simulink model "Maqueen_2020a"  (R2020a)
settings: Solver=VariableStepAuto  StartTime=0.0  StopTime=2  RelTol=1e-3
model workspace: external: MAT-File (data not in the file)
undefined symbols (not defined in the file or in its folder): deg, kg, m, mm, N, rad, s, smiData, X, Y, Z
libraries: sm_lib x459, fl_lib x12, nesl_utility x10
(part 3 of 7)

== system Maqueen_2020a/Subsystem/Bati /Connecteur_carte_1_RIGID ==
  ReferenceFrame : sm_lib/Frames and Transforms/Reference Frame
  Solid : sm_lib/Body Elements/File Solid  ExtGeomFileName=Connecteur carte_Defaut_sldprt.STL  UnitType=Custom  ExtGeomFileUnits=mm  StepReaderType=HEX  ExportConvexHullGeometry=off  InertiaType=Custom  Mass=smiData.Solid(28).mass  MassUnits=kg  CenterOfMass=smiData.Solid(28).CoM  CenterOfMassUnits=mm  MomentsOfInertia=smiData.Solid(28).MoI  MomentsOfInertiaUnits=kg*mm^2  ProductsOfInertia=smiData.Solid(28).PoI  ProductsOfInertiaUnits=kg*mm^2  BasedOnType=Density  Density=1000  DensityUnits=kg/m^3  DoExposeReferenceFrame=on  SerializedFrames=<Frames/>  GraphicType=FromGeometry  MarkerShape=Sphere  MarkerSize=10  GraphicVisPropType=SimpleVisualProperties  GraphicDiffuseColor=smiData.Solid(28).color  GraphicSpecularColor=[0.5 0.5 0.5 1.0]  GraphicAmbientColor=[0.15 0.15 0.15 1.0]  GraphicEmissiveColor=[0.0 0.0 0.0 1.0]  GraphicShininess=75  GraphicOpacity=smiData.Solid(28).opacity
  Transform : sm_lib/Frames and Transforms/Rigid Transform  TranslationMethod=Cartesian  TranslationStandardOffset=0  TranslationLengthUnit=mm  TranslationStandardAxis=+Z  TranslationCartesianOffset=smiData.RigidTransform(4).translation  TranslationROffset=0  TranslationROffsetUnits=m  TranslationZOffset=0  TranslationZOffsetUnits=m  TranslationThetaOffset=0  TranslationThetaOffsetUnits=deg  RotationMethod=ArbitraryAxis  RotationAngleUnits=rad  RotationStandardAxis=+Z  RotationAngle=smiData.RigidTransform(4).angle  RotationArbitraryAxis=smiData.RigidTransform(4).axis  FollAlignAxisA=+X  BaseAlignAxisA=+Y  FollAlignAxisB=+Y  BaseAlignAxisB=+Z  RotationSequenceAxes=FollowerAxes  RotationSequence=XYX  RotationSequenceAngles=[0 0 0]  RotationSequenceAnglesUnits=deg  RotationMatrix=[1 0 0; 0 1 0; 0 0 1]
  Transform1 : sm_lib/Frames and Transforms/Rigid Transform  TranslationMethod=Cartesian  TranslationStandardOffset=0  TranslationLengthUnit=mm  TranslationStandardAxis=+Z  TranslationCartesianOffset=smiData.RigidTransform(5).translation  TranslationROffset=0  TranslationROffsetUnits=m  TranslationZOffset=0  TranslationZOffsetUnits=m  TranslationThetaOffset=0  TranslationThetaOffsetUnits=deg  RotationMethod=ArbitraryAxis  RotationAngleUnits=rad  RotationStandardAxis=+Z  RotationAngle=smiData.RigidTransform(5).angle  RotationArbitraryAxis=smiData.RigidTransform(5).axis  FollAlignAxisA=+X  BaseAlignAxisA=+Y  FollAlignAxisB=+Y  BaseAlignAxisB=+Z  RotationSequenceAxes=FollowerAxes  RotationSequence=XYX  RotationSequenceAngles=[0 0 0]  RotationSequenceAnglesUnits=deg  RotationMatrix=[1 0 0; 0 1 0; 0 0 1]
  F : PMIOPort  Side=Left
  F1 : PMIOPort  Port=2  Side=Left
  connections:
  ReferenceFrame/RConn1 -- Transform/LConn1 -- Transform1/LConn1 -- Solid/RConn1
  Transform/RConn1 -- F/RConn1
  Transform1/RConn1 -- F1/RConn1

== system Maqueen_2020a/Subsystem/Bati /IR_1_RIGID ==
  ReferenceFrame : sm_lib/Frames and Transforms/Reference Frame
  Solid : sm_lib/Body Elements/File Solid  ExtGeomFileName=IR_Defaut_sldprt.STL  UnitType=Custom  ExtGeomFileUnits=mm  StepReaderType=HEX  ExportConvexHullGeometry=off  InertiaType=Custom  Mass=smiData.Solid(32).mass  MassUnits=kg  CenterOfMass=smiData.Solid(32).CoM  CenterOfMassUnits=mm  MomentsOfInertia=smiData.Solid(32).MoI  MomentsOfInertiaUnits=kg*mm^2  ProductsOfInertia=smiData.Solid(32).PoI  ProductsOfInertiaUnits=kg*mm^2  BasedOnType=Density  Density=1000  DensityUnits=kg/m^3  DoExposeReferenceFrame=on  SerializedFrames=<Frames/>  GraphicType=FromGeometry  MarkerShape=Sphere  MarkerSize=10  GraphicVisPropType=SimpleVisualProperties  GraphicDiffuseColor=smiData.Solid(32).color  GraphicSpecularColor=[0.5 0.5 0.5 1.0]  GraphicAmbientColor=[0.15 0.15 0.15 1.0]  GraphicEmissiveColor=[0.0 0.0 0.0 1.0]  GraphicShininess=75  GraphicOpacity=smiData.Solid(32).opacity
  Transform : sm_lib/Frames and Transforms/Rigid Transform  TranslationMethod=Cartesian  TranslationStandardOffset=0  TranslationLengthUnit=mm  TranslationStandardAxis=+Z  TranslationCartesianOffset=smiData.RigidTransform(10).translation  TranslationROffset=0  TranslationROffsetUnits=m  TranslationZOffset=0  TranslationZOffsetUnits=m  TranslationThetaOffset=0  TranslationThetaOffsetUnits=deg  RotationMethod=ArbitraryAxis  RotationAngleUnits=rad  RotationStandardAxis=+Z  RotationAngle=smiData.RigidTransform(10).angle  RotationArbitraryAxis=smiData.RigidTransform(10).axis  FollAlignAxisA=+X  BaseAlignAxisA=+Y  FollAlignAxisB=+Y  BaseAlignAxisB=+Z  RotationSequenceAxes=FollowerAxes  RotationSequence=XYX  RotationSequenceAngles=[0 0 0]  RotationSequenceAnglesUnits=deg  RotationMatrix=[1 0 0; 0 1 0; 0 0 1]
  F : PMIOPort  Side=Left
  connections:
  ReferenceFrame/RConn1 -- Solid/RConn1 -- Transform/LConn1
  Transform/RConn1 -- F/RConn1

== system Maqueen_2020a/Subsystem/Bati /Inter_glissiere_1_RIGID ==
  ReferenceFrame : sm_lib/Frames and Transforms/Reference Frame
  Solid : sm_lib/Body Elements/File Solid  ExtGeomFileName=Inter_glissiere_Defaut_sldprt.STL  UnitType=Custom  ExtGeomFileUnits=mm  StepReaderType=HEX  ExportConvexHullGeometry=off  InertiaType=Custom  Mass=smiData.Solid(1).mass  MassUnits=kg  CenterOfMass=smiData.Solid(1).CoM  CenterOfMassUnits=mm  MomentsOfInertia=smiData.Solid(1).MoI  MomentsOfInertiaUnits=kg*mm^2  ProductsOfInertia=smiData.Solid(1).PoI  ProductsOfInertiaUnits=kg*mm^2  BasedOnType=Density  Density=1000  DensityUnits=kg/m^3  DoExposeReferenceFrame=on  SerializedFrames=<Frames/>  GraphicType=FromGeometry  MarkerShape=Sphere  MarkerSize=10  GraphicVisPropType=SimpleVisualProperties  GraphicDiffuseColor=smiData.Solid(1).color  GraphicSpecularColor=[0.5 0.5 0.5 1.0]  GraphicAmbientColor=[0.15 0.15 0.15 1.0]  GraphicEmissiveColor=[0.0 0.0 0.0 1.0]  GraphicShininess=75  GraphicOpacity=smiData.Solid(1).opacity
  Transform : sm_lib/Frames and Transforms/Rigid Transform  TranslationMethod=Cartesian  TranslationStandardOffset=0  TranslationLengthUnit=mm  TranslationStandardAxis=+Z  TranslationCartesianOffset=smiData.RigidTransform(12).translation  TranslationROffset=0  TranslationROffsetUnits=m  TranslationZOffset=0  TranslationZOffsetUnits=m  TranslationThetaOffset=0  TranslationThetaOffsetUnits=deg  RotationMethod=ArbitraryAxis  RotationAngleUnits=rad  RotationStandardAxis=+Z  RotationAngle=smiData.RigidTransform(12).angle  RotationArbitraryAxis=smiData.RigidTransform(12).axis  FollAlignAxisA=+X  BaseAlignAxisA=+Y  FollAlignAxisB=+Y  BaseAlignAxisB=+Z  RotationSequenceAxes=FollowerAxes  RotationSequence=XYX  RotationSequenceAngles=[0 0 0]  RotationSequenceAnglesUnits=deg  RotationMatrix=[1 0 0; 0 1 0; 0 0 1]
  F : PMIOPort  Side=Left
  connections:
  ReferenceFrame/RConn1 -- Solid/RConn1 -- Transform/LConn1
  Transform/RConn1 -- F/RConn1

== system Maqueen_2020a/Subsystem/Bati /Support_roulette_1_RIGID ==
  ReferenceFrame : sm_lib/Frames and Transforms/Reference Frame
  Rouleau_1_RIGID : Subsystem
  Support_roulette_1_RIGID : Subsystem
  Transform : sm_lib/Frames and Transforms/Rigid Transform  TranslationMethod=Cartesian  TranslationStandardOffset=0  TranslationLengthUnit=mm  TranslationStandardAxis=+Z  TranslationCartesianOffset=smiData.RigidTransform(8).translation  TranslationROffset=0  TranslationROffsetUnits=m  TranslationZOffset=0  TranslationZOffsetUnits=m  TranslationThetaOffset=0  TranslationThetaOffsetUnits=deg  RotationMethod=ArbitraryAxis  RotationAngleUnits=rad  RotationStandardAxis=+Z  RotationAngle=smiData.RigidTransform(8).angle  RotationArbitraryAxis=smiData.RigidTransform(8).axis  FollAlignAxisA=+X  BaseAlignAxisA=+Y  FollAlignAxisB=+Y  BaseAlignAxisB=+Z  RotationSequenceAxes=FollowerAxes  RotationSequence=XYX  RotationSequenceAngles=[0 0 0]  RotationSequenceAnglesUnits=deg  RotationMatrix=[1 0 0; 0 1 0; 0 0 1]
  Transform1 : sm_lib/Frames and Transforms/Rigid Transform  TranslationMethod=Cartesian  TranslationStandardOffset=0  TranslationLengthUnit=mm  TranslationStandardAxis=+Z  TranslationCartesianOffset=smiData.RigidTransform(159).translation  TranslationROffset=0  TranslationROffsetUnits=m  TranslationZOffset=0  TranslationZOffsetUnits=m  TranslationThetaOffset=0  TranslationThetaOffsetUnits=deg  RotationMethod=ArbitraryAxis  RotationAngleUnits=rad  RotationStandardAxis=+Z  RotationAngle=smiData.RigidTransform(159).angle  RotationArbitraryAxis=smiData.RigidTransform(159).axis  FollAlignAxisA=+X  BaseAlignAxisA=+Y  FollAlignAxisB=+Y  BaseAlignAxisB=+Z  RotationSequenceAxes=FollowerAxes  RotationSequence=XYX  RotationSequenceAngles=[0 0 0]  RotationSequenceAnglesUnits=deg  RotationMatrix=[1 0 0; 0 1 0; 0 0 1]
  Transform2 : sm_lib/Frames and Transforms/Rigid Transform  TranslationMethod=Cartesian  TranslationStandardOffset=0  TranslationLengthUnit=mm  TranslationStandardAxis=+Z  TranslationCartesianOffset=smiData.RigidTransform(160).translation  TranslationROffset=0  TranslationROffsetUnits=m  TranslationZOffset=0  TranslationZOffsetUnits=m  TranslationThetaOffset=0  TranslationThetaOffsetUnits=deg  RotationMethod=ArbitraryAxis  RotationAngleUnits=rad  RotationStandardAxis=+Z  RotationAngle=smiData.RigidTransform(160).angle  RotationArbitraryAxis=smiData.RigidTransform(160).axis  FollAlignAxisA=+X  BaseAlignAxisA=+Y  FollAlignAxisB=+Y  BaseAlignAxisB=+Z  RotationSequenceAxes=FollowerAxes  RotationSequence=XYX  RotationSequenceAngles=[0 0 0]  RotationSequenceAnglesUnits=deg  RotationMatrix=[1 0 0; 0 1 0; 0 0 1]
  F : PMIOPort  Side=Left
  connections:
  ReferenceFrame/RConn1 -- Transform/LConn1 -- Transform1/LConn1 -- Transform2/LConn1
  Transform/RConn1 -- F/RConn1
  Support_roulette_1_RIGID/LConn1 -- Transform1/RConn1
  Rouleau_1_RIGID/LConn1 -- Transform2/RConn1

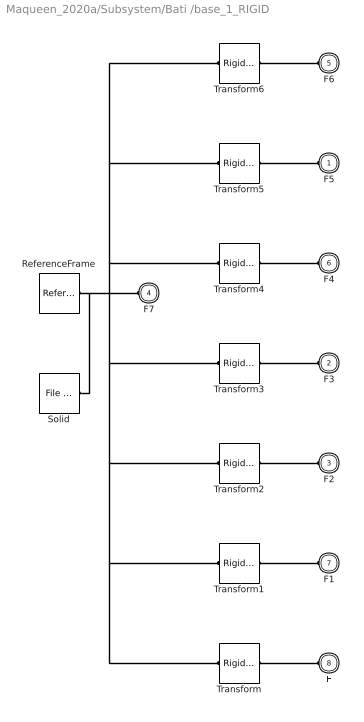
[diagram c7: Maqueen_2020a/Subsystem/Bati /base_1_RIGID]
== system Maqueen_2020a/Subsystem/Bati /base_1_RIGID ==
  ReferenceFrame : sm_lib/Frames and Transforms/Reference Frame
  Solid : sm_lib/Body Elements/File Solid  ExtGeomFileName=base_Defaut_sldprt.STL  UnitType=Custom  ExtGeomFileUnits=mm  StepReaderType=HEX  ExportConvexHullGeometry=off  InertiaType=Custom  Mass=smiData.Solid(29).mass  MassUnits=kg  CenterOfMass=smiData.Solid(29).CoM  CenterOfMassUnits=mm  MomentsOfInertia=smiData.Solid(29).MoI  MomentsOfInertiaUnits=kg*mm^2  ProductsOfInertia=smiData.Solid(29).PoI  ProductsOfInertiaUnits=kg*mm^2  BasedOnType=Density  Density=1000  DensityUnits=kg/m^3  DoExposeReferenceFrame=on  SerializedFrames=<Frames/>  GraphicType=FromGeometry  MarkerShape=Sphere  MarkerSize=10  GraphicVisPropType=SimpleVisualProperties  GraphicDiffuseColor=smiData.Solid(29).color  GraphicSpecularColor=[0.5 0.5 0.5 1.0]  GraphicAmbientColor=[0.15 0.15 0.15 1.0]  GraphicEmissiveColor=[0.0 0.0 0.0 1.0]  GraphicShininess=75  GraphicOpacity=smiData.Solid(29).opacity
  Transform : sm_lib/Frames and Transforms/Rigid Transform  TranslationMethod=Cartesian  TranslationStandardOffset=0  TranslationLengthUnit=mm  TranslationStandardAxis=+Z  TranslationCartesianOffset=smiData.RigidTransform(3).translation  TranslationROffset=0  TranslationROffsetUnits=m  TranslationZOffset=0  TranslationZOffsetUnits=m  TranslationThetaOffset=0  TranslationThetaOffsetUnits=deg  RotationMethod=ArbitraryAxis  RotationAngleUnits=rad  RotationStandardAxis=+Z  RotationAngle=smiData.RigidTransform(3).angle  RotationArbitraryAxis=smiData.RigidTransform(3).axis  FollAlignAxisA=+X  BaseAlignAxisA=+Y  FollAlignAxisB=+Y  BaseAlignAxisB=+Z  RotationSequenceAxes=FollowerAxes  RotationSequence=XYX  RotationSequenceAngles=[0 0 0]  RotationSequenceAnglesUnits=deg  RotationMatrix=[1 0 0; 0 1 0; 0 0 1]
  Transform1 : sm_lib/Frames and Transforms/Rigid Transform  TranslationMethod=Cartesian  TranslationStandardOffset=0  TranslationLengthUnit=mm  TranslationStandardAxis=+Z  TranslationCartesianOffset=smiData.RigidTransform(7).translation  TranslationROffset=0  TranslationROffsetUnits=m  TranslationZOffset=0  TranslationZOffsetUnits=m  TranslationThetaOffset=0  TranslationThetaOffsetUnits=deg  RotationMethod=ArbitraryAxis  RotationAngleUnits=rad  RotationStandardAxis=+Z  RotationAngle=smiData.RigidTransform(7).angle  RotationArbitraryAxis=smiData.RigidTransform(7).axis  FollAlignAxisA=+X  BaseAlignAxisA=+Y  FollAlignAxisB=+Y  BaseAlignAxisB=+Z  RotationSequenceAxes=FollowerAxes  RotationSequence=XYX  RotationSequenceAngles=[0 0 0]  RotationSequenceAnglesUnits=deg  RotationMatrix=[1 0 0; 0 1 0; 0 0 1]
  Transform2 : sm_lib/Frames and Transforms/Rigid Transform  TranslationMethod=Cartesian  TranslationStandardOffset=0  TranslationLengthUnit=mm  TranslationStandardAxis=+Z  TranslationCartesianOffset=smiData.RigidTransform(9).translation  TranslationROffset=0  TranslationROffsetUnits=m  TranslationZOffset=0  TranslationZOffsetUnits=m  TranslationThetaOffset=0  TranslationThetaOffsetUnits=deg  RotationMethod=ArbitraryAxis  RotationAngleUnits=rad  RotationStandardAxis=+Z  RotationAngle=smiData.RigidTransform(9).angle  RotationArbitraryAxis=smiData.RigidTransform(9).axis  FollAlignAxisA=+X  BaseAlignAxisA=+Y  FollAlignAxisB=+Y  BaseAlignAxisB=+Z  RotationSequenceAxes=FollowerAxes  RotationSequence=XYX  RotationSequenceAngles=[0 0 0]  RotationSequenceAnglesUnits=deg  RotationMatrix=[1 0 0; 0 1 0; 0 0 1]
  Transform3 : sm_lib/Frames and Transforms/Rigid Transform  TranslationMethod=Cartesian  TranslationStandardOffset=0  TranslationLengthUnit=mm  TranslationStandardAxis=+Z  TranslationCartesianOffset=smiData.RigidTransform(11).translation  TranslationROffset=0  TranslationROffsetUnits=m  TranslationZOffset=0  TranslationZOffsetUnits=m  TranslationThetaOffset=0  TranslationThetaOffsetUnits=deg  RotationMethod=ArbitraryAxis  RotationAngleUnits=rad  RotationStandardAxis=+Z  RotationAngle=smiData.RigidTransform(11).angle  RotationArbitraryAxis=smiData.RigidTransform(11).axis  FollAlignAxisA=+X  BaseAlignAxisA=+Y  FollAlignAxisB=+Y  BaseAlignAxisB=+Z  RotationSequenceAxes=FollowerAxes  RotationSequence=XYX  RotationSequenceAngles=[0 0 0]  RotationSequenceAnglesUnits=deg  RotationMatrix=[1 0 0; 0 1 0; 0 0 1]
  Transform4 : sm_lib/Frames and Transforms/Rigid Transform  TranslationMethod=Cartesian  TranslationStandardOffset=0  TranslationLengthUnit=mm  TranslationStandardAxis=+Z  TranslationCartesianOffset=smiData.RigidTransform(13).translation  TranslationROffset=0  TranslationROffsetUnits=m  TranslationZOffset=0  TranslationZOffsetUnits=m  TranslationThetaOffset=0  TranslationThetaOffsetUnits=deg  RotationMethod=ArbitraryAxis  RotationAngleUnits=rad  RotationStandardAxis=+Z  RotationAngle=smiData.RigidTransform(13).angle  RotationArbitraryAxis=smiData.RigidTransform(13).axis  FollAlignAxisA=+X  BaseAlignAxisA=+Y  FollAlignAxisB=+Y  BaseAlignAxisB=+Z  RotationSequenceAxes=FollowerAxes  RotationSequence=XYX  RotationSequenceAngles=[0 0 0]  RotationSequenceAnglesUnits=deg  RotationMatrix=[1 0 0; 0 1 0; 0 0 1]
  Transform5 : sm_lib/Frames and Transforms/Rigid Transform  TranslationMethod=Cartesian  TranslationStandardOffset=0  TranslationLengthUnit=mm  TranslationStandardAxis=+Z  TranslationCartesianOffset=smiData.RigidTransform(17).translation  TranslationROffset=0  TranslationROffsetUnits=m  TranslationZOffset=0  TranslationZOffsetUnits=m  TranslationThetaOffset=0  TranslationThetaOffsetUnits=deg  RotationMethod=ArbitraryAxis  RotationAngleUnits=rad  RotationStandardAxis=+Z  RotationAngle=smiData.RigidTransform(17).angle  RotationArbitraryAxis=smiData.RigidTransform(17).axis  FollAlignAxisA=+X  BaseAlignAxisA=+Y  FollAlignAxisB=+Y  BaseAlignAxisB=+Z  RotationSequenceAxes=FollowerAxes  RotationSequence=XYX  RotationSequenceAngles=[0 0 0]  RotationSequenceAnglesUnits=deg  RotationMatrix=[1 0 0; 0 1 0; 0 0 1]
  Transform6 : sm_lib/Frames and Transforms/Rigid Transform  TranslationMethod=Cartesian  TranslationStandardOffset=0  TranslationLengthUnit=mm  TranslationStandardAxis=+Z  TranslationCartesianOffset=smiData.RigidTransform(21).translation  TranslationROffset=0  TranslationROffsetUnits=m  TranslationZOffset=0  TranslationZOffsetUnits=m  TranslationThetaOffset=0  TranslationThetaOffsetUnits=deg  RotationMethod=ArbitraryAxis  RotationAngleUnits=rad  RotationStandardAxis=+Z  RotationAngle=smiData.RigidTransform(21).angle  RotationArbitraryAxis=smiData.RigidTransform(21).axis  FollAlignAxisA=+X  BaseAlignAxisA=+Y  FollAlignAxisB=+Y  BaseAlignAxisB=+Z  RotationSequenceAxes=FollowerAxes  RotationSequence=XYX  RotationSequenceAngles=[0 0 0]  RotationSequenceAnglesUnits=deg  RotationMatrix=[1 0 0; 0 1 0; 0 0 1]
  F5 : PMIOPort  Side=Left
  F3 : PMIOPort  Port=2  Side=Left
  F2 : PMIOPort  Port=3  Side=Left
  F7 : PMIOPort  Port=4  Side=Left
  F6 : PMIOPort  Port=5  Side=Left
  F4 : PMIOPort  Port=6  Side=Left
  F1 : PMIOPort  Port=7  Side=Left
  F : PMIOPort  Port=8  Side=Left
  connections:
  ReferenceFrame/RConn1 -- Transform/LConn1 -- Transform1/LConn1 -- Transform2/LConn1 -- Transform3/LConn1 -- Transform5/LConn1 -- Transform6/LConn1 -- Transform4/LConn1 -- F7/RConn1 -- Solid/RConn1
  Transform/RConn1 -- F/RConn1
  Transform1/RConn1 -- F1/RConn1
  Transform2/RConn1 -- F2/RConn1
  Transform3/RConn1 -- F3/RConn1
  Transform4/RConn1 -- F4/RConn1
  Transform5/RConn1 -- F5/RConn1
  Transform6/RConn1 -- F6/RConn1

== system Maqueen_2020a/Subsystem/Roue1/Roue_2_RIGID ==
  Jante_1_RIGID : Subsystem
  Pneu_1_RIGID : Subsystem
  ReferenceFrame : sm_lib/Frames and Transforms/Reference Frame
  Transform : sm_lib/Frames and Transforms/Rigid Transform  TranslationMethod=Cartesian  TranslationStandardOffset=0  TranslationLengthUnit=mm  TranslationStandardAxis=+Z  TranslationCartesianOffset=smiData.RigidTransform(15).translation  TranslationROffset=0  TranslationROffsetUnits=m  TranslationZOffset=0  TranslationZOffsetUnits=m  TranslationThetaOffset=0  TranslationThetaOffsetUnits=deg  RotationMethod=ArbitraryAxis  RotationAngleUnits=rad  RotationStandardAxis=+Z  RotationAngle=smiData.RigidTransform(15).angle  RotationArbitraryAxis=smiData.RigidTransform(15).axis  FollAlignAxisA=+X  BaseAlignAxisA=+Y  FollAlignAxisB=+Y  BaseAlignAxisB=+Z  RotationSequenceAxes=FollowerAxes  RotationSequence=XYX  RotationSequenceAngles=[0 0 0]  RotationSequenceAnglesUnits=deg  RotationMatrix=[1 0 0; 0 1 0; 0 0 1]
  Transform1 : sm_lib/Frames and Transforms/Rigid Transform  TranslationMethod=Cartesian  TranslationStandardOffset=0  TranslationLengthUnit=mm  TranslationStandardAxis=+Z  TranslationCartesianOffset=smiData.RigidTransform(23).translation  TranslationROffset=0  TranslationROffsetUnits=m  TranslationZOffset=0  TranslationZOffsetUnits=m  TranslationThetaOffset=0  TranslationThetaOffsetUnits=deg  RotationMethod=ArbitraryAxis  RotationAngleUnits=rad  RotationStandardAxis=+Z  RotationAngle=smiData.RigidTransform(23).angle  RotationArbitraryAxis=smiData.RigidTransform(23).axis  FollAlignAxisA=+X  BaseAlignAxisA=+Y  FollAlignAxisB=+Y  BaseAlignAxisB=+Z  RotationSequenceAxes=FollowerAxes  RotationSequence=XYX  RotationSequenceAngles=[0 0 0]  RotationSequenceAnglesUnits=deg  RotationMatrix=[1 0 0; 0 1 0; 0 0 1]
  Transform2 : sm_lib/Frames and Transforms/Rigid Transform  TranslationMethod=Cartesian  TranslationStandardOffset=0  TranslationLengthUnit=mm  TranslationStandardAxis=+Z  TranslationCartesianOffset=smiData.RigidTransform(24).translation  TranslationROffset=0  TranslationROffsetUnits=m  TranslationZOffset=0  TranslationZOffsetUnits=m  TranslationThetaOffset=0  TranslationThetaOffsetUnits=deg  RotationMethod=ArbitraryAxis  RotationAngleUnits=rad  RotationStandardAxis=+Z  RotationAngle=smiData.RigidTransform(24).angle  RotationArbitraryAxis=smiData.RigidTransform(24).axis  FollAlignAxisA=+X  BaseAlignAxisA=+Y  FollAlignAxisB=+Y  BaseAlignAxisB=+Z  RotationSequenceAxes=FollowerAxes  RotationSequence=XYX  RotationSequenceAngles=[0 0 0]  RotationSequenceAnglesUnits=deg  RotationMatrix=[1 0 0; 0 1 0; 0 0 1]
  F : PMIOPort  Side=Right
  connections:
  ReferenceFrame/RConn1 -- Transform/LConn1 -- Transform1/LConn1 -- Transform2/LConn1
  Transform/RConn1 -- F/RConn1
  Pneu_1_RIGID/LConn1 -- Transform1/RConn1
  Jante_1_RIGID/LConn1 -- Transform2/RConn1

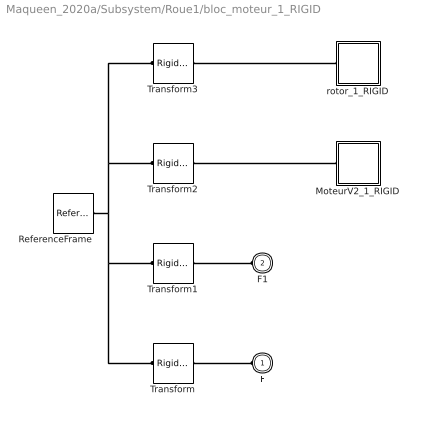
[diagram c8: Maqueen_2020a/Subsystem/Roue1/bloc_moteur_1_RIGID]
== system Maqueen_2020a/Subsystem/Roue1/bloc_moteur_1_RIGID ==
  MoteurV2_1_RIGID : Subsystem
  ReferenceFrame : sm_lib/Frames and Transforms/Reference Frame
  Transform : sm_lib/Frames and Transforms/Rigid Transform  TranslationMethod=Cartesian  TranslationStandardOffset=0  TranslationLengthUnit=mm  TranslationStandardAxis=+Z  TranslationCartesianOffset=smiData.RigidTransform(16).translation  TranslationROffset=0  TranslationROffsetUnits=m  TranslationZOffset=0  TranslationZOffsetUnits=m  TranslationThetaOffset=0  TranslationThetaOffsetUnits=deg  RotationMethod=ArbitraryAxis  RotationAngleUnits=rad  RotationStandardAxis=+Z  RotationAngle=smiData.RigidTransform(16).angle  RotationArbitraryAxis=smiData.RigidTransform(16).axis  FollAlignAxisA=+X  BaseAlignAxisA=+Y  FollAlignAxisB=+Y  BaseAlignAxisB=+Z  RotationSequenceAxes=FollowerAxes  RotationSequence=XYX  RotationSequenceAngles=[0 0 0]  RotationSequenceAnglesUnits=deg  RotationMatrix=[1 0 0; 0 1 0; 0 0 1]
  Transform1 : sm_lib/Frames and Transforms/Rigid Transform  TranslationMethod=Cartesian  TranslationStandardOffset=0  TranslationLengthUnit=mm  TranslationStandardAxis=+Z  TranslationCartesianOffset=smiData.RigidTransform(18).translation  TranslationROffset=0  TranslationROffsetUnits=m  TranslationZOffset=0  TranslationZOffsetUnits=m  TranslationThetaOffset=0  TranslationThetaOffsetUnits=deg  RotationMethod=ArbitraryAxis  RotationAngleUnits=rad  RotationStandardAxis=+Z  RotationAngle=smiData.RigidTransform(18).angle  RotationArbitraryAxis=smiData.RigidTransform(18).axis  FollAlignAxisA=+X  BaseAlignAxisA=+Y  FollAlignAxisB=+Y  BaseAlignAxisB=+Z  RotationSequenceAxes=FollowerAxes  RotationSequence=XYX  RotationSequenceAngles=[0 0 0]  RotationSequenceAnglesUnits=deg  RotationMatrix=[1 0 0; 0 1 0; 0 0 1]
  Transform2 : sm_lib/Frames and Transforms/Rigid Transform  TranslationMethod=Cartesian  TranslationStandardOffset=0  TranslationLengthUnit=mm  TranslationStandardAxis=+Z  TranslationCartesianOffset=smiData.RigidTransform(25).translation  TranslationROffset=0  TranslationROffsetUnits=m  TranslationZOffset=0  TranslationZOffsetUnits=m  TranslationThetaOffset=0  TranslationThetaOffsetUnits=deg  RotationMethod=ArbitraryAxis  RotationAngleUnits=rad  RotationStandardAxis=+Z  RotationAngle=smiData.RigidTransform(25).angle  RotationArbitraryAxis=smiData.RigidTransform(25).axis  FollAlignAxisA=+X  BaseAlignAxisA=+Y  FollAlignAxisB=+Y  BaseAlignAxisB=+Z  RotationSequenceAxes=FollowerAxes  RotationSequence=XYX  RotationSequenceAngles=[0 0 0]  RotationSequenceAnglesUnits=deg  RotationMatrix=[1 0 0; 0 1 0; 0 0 1]
  Transform3 : sm_lib/Frames and Transforms/Rigid Transform  TranslationMethod=Cartesian  TranslationStandardOffset=0  TranslationLengthUnit=mm  TranslationStandardAxis=+Z  TranslationCartesianOffset=smiData.RigidTransform(26).translation  TranslationROffset=0  TranslationROffsetUnits=m  TranslationZOffset=0  TranslationZOffsetUnits=m  TranslationThetaOffset=0  TranslationThetaOffsetUnits=deg  RotationMethod=ArbitraryAxis  RotationAngleUnits=rad  RotationStandardAxis=+Z  RotationAngle=smiData.RigidTransform(26).angle  RotationArbitraryAxis=smiData.RigidTransform(26).axis  FollAlignAxisA=+X  BaseAlignAxisA=+Y  FollAlignAxisB=+Y  BaseAlignAxisB=+Z  RotationSequenceAxes=FollowerAxes  RotationSequence=XYX  RotationSequenceAngles=[0 0 0]  RotationSequenceAnglesUnits=deg  RotationMatrix=[1 0 0; 0 1 0; 0 0 1]
  rotor_1_RIGID : Subsystem
  F : PMIOPort  Side=Left
  F1 : PMIOPort  Port=2  Side=Left
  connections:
  ReferenceFrame/RConn1 -- Transform/LConn1 -- Transform1/LConn1 -- Transform2/LConn1 -- Transform3/LConn1
  Transform/RConn1 -- F/RConn1
  Transform1/RConn1 -- F1/RConn1
  MoteurV2_1_RIGID/LConn1 -- Transform2/RConn1
  Transform3/RConn1 -- rotor_1_RIGID/LConn1

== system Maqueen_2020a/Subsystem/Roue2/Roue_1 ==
  Jante_1_RIGID : Subsystem
  Pneu_1_RIGID : Subsystem
  ReferenceFrame : sm_lib/Frames and Transforms/Reference Frame
  Transform : sm_lib/Frames and Transforms/Rigid Transform  TranslationMethod=Cartesian  TranslationStandardOffset=0  TranslationLengthUnit=mm  TranslationStandardAxis=+Z  TranslationCartesianOffset=smiData.RigidTransform(162).translation  TranslationROffset=0  TranslationROffsetUnits=m  TranslationZOffset=0  TranslationZOffsetUnits=m  TranslationThetaOffset=0  TranslationThetaOffsetUnits=deg  RotationMethod=ArbitraryAxis  RotationAngleUnits=rad  RotationStandardAxis=+Z  RotationAngle=smiData.RigidTransform(162).angle  RotationArbitraryAxis=smiData.RigidTransform(162).axis  FollAlignAxisA=+X  BaseAlignAxisA=+Y  FollAlignAxisB=+Y  BaseAlignAxisB=+Z  RotationSequenceAxes=FollowerAxes  RotationSequence=XYX  RotationSequenceAngles=[0 0 0]  RotationSequenceAnglesUnits=deg  RotationMatrix=[1 0 0; 0 1 0; 0 0 1]
  F : PMIOPort  Side=Right
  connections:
  Jante_1_RIGID/LConn3 -- Pneu_1_RIGID/LConn1
  Jante_1_RIGID/LConn2 -- F/RConn1
  Jante_1_RIGID/LConn1 -- Transform/RConn1
  ReferenceFrame/RConn1 -- Transform/LConn1

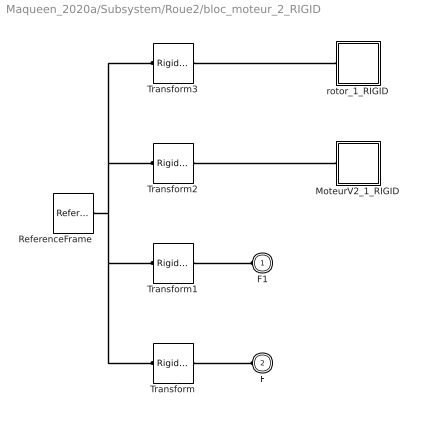
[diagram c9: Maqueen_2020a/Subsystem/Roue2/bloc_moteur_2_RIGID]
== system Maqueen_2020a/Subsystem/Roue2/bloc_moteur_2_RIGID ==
  MoteurV2_1_RIGID : Subsystem
  ReferenceFrame : sm_lib/Frames and Transforms/Reference Frame
  Transform : sm_lib/Frames and Transforms/Rigid Transform  TranslationMethod=Cartesian  TranslationStandardOffset=0  TranslationLengthUnit=mm  TranslationStandardAxis=+Z  TranslationCartesianOffset=smiData.RigidTransform(20).translation  TranslationROffset=0  TranslationROffsetUnits=m  TranslationZOffset=0  TranslationZOffsetUnits=m  TranslationThetaOffset=0  TranslationThetaOffsetUnits=deg  RotationMethod=ArbitraryAxis  RotationAngleUnits=rad  RotationStandardAxis=+Z  RotationAngle=smiData.RigidTransform(20).angle  RotationArbitraryAxis=smiData.RigidTransform(20).axis  FollAlignAxisA=+X  BaseAlignAxisA=+Y  FollAlignAxisB=+Y  BaseAlignAxisB=+Z  RotationSequenceAxes=FollowerAxes  RotationSequence=XYX  RotationSequenceAngles=[0 0 0]  RotationSequenceAnglesUnits=deg  RotationMatrix=[1 0 0; 0 1 0; 0 0 1]
  Transform1 : sm_lib/Frames and Transforms/Rigid Transform  TranslationMethod=Cartesian  TranslationStandardOffset=0  TranslationLengthUnit=mm  TranslationStandardAxis=+Z  TranslationCartesianOffset=smiData.RigidTransform(22).translation  TranslationROffset=0  TranslationROffsetUnits=m  TranslationZOffset=0  TranslationZOffsetUnits=m  TranslationThetaOffset=0  TranslationThetaOffsetUnits=deg  RotationMethod=ArbitraryAxis  RotationAngleUnits=rad  RotationStandardAxis=+Z  RotationAngle=smiData.RigidTransform(22).angle  RotationArbitraryAxis=smiData.RigidTransform(22).axis  FollAlignAxisA=+X  BaseAlignAxisA=+Y  FollAlignAxisB=+Y  BaseAlignAxisB=+Z  RotationSequenceAxes=FollowerAxes  RotationSequence=XYX  RotationSequenceAngles=[0 0 0]  RotationSequenceAnglesUnits=deg  RotationMatrix=[1 0 0; 0 1 0; 0 0 1]
  Transform2 : sm_lib/Frames and Transforms/Rigid Transform  TranslationMethod=Cartesian  TranslationStandardOffset=0  TranslationLengthUnit=mm  TranslationStandardAxis=+Z  TranslationCartesianOffset=smiData.RigidTransform(27).translation  TranslationROffset=0  TranslationROffsetUnits=m  TranslationZOffset=0  TranslationZOffsetUnits=m  TranslationThetaOffset=0  TranslationThetaOffsetUnits=deg  RotationMethod=ArbitraryAxis  RotationAngleUnits=rad  RotationStandardAxis=+Z  RotationAngle=smiData.RigidTransform(27).angle  RotationArbitraryAxis=smiData.RigidTransform(27).axis  FollAlignAxisA=+X  BaseAlignAxisA=+Y  FollAlignAxisB=+Y  BaseAlignAxisB=+Z  RotationSequenceAxes=FollowerAxes  RotationSequence=XYX  RotationSequenceAngles=[0 0 0]  RotationSequenceAnglesUnits=deg  RotationMatrix=[1 0 0; 0 1 0; 0 0 1]
  Transform3 : sm_lib/Frames and Transforms/Rigid Transform  TranslationMethod=Cartesian  TranslationStandardOffset=0  TranslationLengthUnit=mm  TranslationStandardAxis=+Z  TranslationCartesianOffset=smiData.RigidTransform(28).translation  TranslationROffset=0  TranslationROffsetUnits=m  TranslationZOffset=0  TranslationZOffsetUnits=m  TranslationThetaOffset=0  TranslationThetaOffsetUnits=deg  RotationMethod=ArbitraryAxis  RotationAngleUnits=rad  RotationStandardAxis=+Z  RotationAngle=smiData.RigidTransform(28).angle  RotationArbitraryAxis=smiData.RigidTransform(28).axis  FollAlignAxisA=+X  BaseAlignAxisA=+Y  FollAlignAxisB=+Y  BaseAlignAxisB=+Z  RotationSequenceAxes=FollowerAxes  RotationSequence=XYX  RotationSequenceAngles=[0 0 0]  RotationSequenceAnglesUnits=deg  RotationMatrix=[1 0 0; 0 1 0; 0 0 1]
  rotor_1_RIGID : Subsystem
  F1 : PMIOPort  Side=Left
  F : PMIOPort  Port=2  Side=Left
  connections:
  ReferenceFrame/RConn1 -- Transform/LConn1 -- Transform1/LConn1 -- Transform2/LConn1 -- Transform3/LConn1
  Transform/RConn1 -- F/RConn1
  Transform1/RConn1 -- F1/RConn1
  MoteurV2_1_RIGID/LConn1 -- Transform2/RConn1
  Transform3/RConn1 -- rotor_1_RIGID/LConn1

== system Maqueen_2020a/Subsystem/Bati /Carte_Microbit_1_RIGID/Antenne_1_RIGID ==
  ReferenceFrame : sm_lib/Frames and Transforms/Reference Frame
  Solid : sm_lib/Body Elements/File Solid  ExtGeomFileName=Antenne_Defaut_sldprt.STL  UnitType=Custom  ExtGeomFileUnits=mm  StepReaderType=HEX  ExportConvexHullGeometry=off  InertiaType=Custom  Mass=smiData.Solid(21).mass  MassUnits=kg  CenterOfMass=smiData.Solid(21).CoM  CenterOfMassUnits=mm  MomentsOfInertia=smiData.Solid(21).MoI  MomentsOfInertiaUnits=kg*mm^2  ProductsOfInertia=smiData.Solid(21).PoI  ProductsOfInertiaUnits=kg*mm^2  BasedOnType=Density  Density=1000  DensityUnits=kg/m^3  DoExposeReferenceFrame=on  SerializedFrames=<Frames/>  GraphicType=FromGeometry  MarkerShape=Sphere  MarkerSize=10  GraphicVisPropType=SimpleVisualProperties  GraphicDiffuseColor=smiData.Solid(21).color  GraphicSpecularColor=[0.5 0.5 0.5 1.0]  GraphicAmbientColor=[0.15 0.15 0.15 1.0]  GraphicEmissiveColor=[0.0 0.0 0.0 1.0]  GraphicShininess=75  GraphicOpacity=smiData.Solid(21).opacity
  F : PMIOPort  Side=Left
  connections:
  ReferenceFrame/RConn1 -- Solid/RConn1 -- F/RConn1

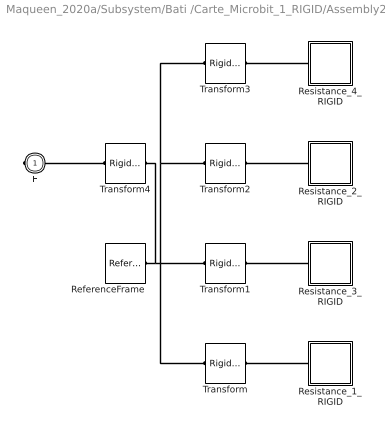
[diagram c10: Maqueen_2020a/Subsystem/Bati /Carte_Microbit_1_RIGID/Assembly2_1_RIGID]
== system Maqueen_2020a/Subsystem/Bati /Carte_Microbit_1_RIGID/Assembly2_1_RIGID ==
  ReferenceFrame : sm_lib/Frames and Transforms/Reference Frame
  Resistance_1_RIGID : Subsystem
  Resistance_2_RIGID : Subsystem
  Resistance_3_RIGID : Subsystem
  Resistance_4_RIGID : Subsystem
  Transform : sm_lib/Frames and Transforms/Rigid Transform  TranslationMethod=Cartesian  TranslationStandardOffset=0  TranslationLengthUnit=mm  TranslationStandardAxis=+Z  TranslationCartesianOffset=smiData.RigidTransform(118).translation  TranslationROffset=0  TranslationROffsetUnits=m  TranslationZOffset=0  TranslationZOffsetUnits=m  TranslationThetaOffset=0  TranslationThetaOffsetUnits=deg  RotationMethod=ArbitraryAxis  RotationAngleUnits=rad  RotationStandardAxis=+Z  RotationAngle=smiData.RigidTransform(118).angle  RotationArbitraryAxis=smiData.RigidTransform(118).axis  FollAlignAxisA=+X  BaseAlignAxisA=+Y  FollAlignAxisB=+Y  BaseAlignAxisB=+Z  RotationSequenceAxes=FollowerAxes  RotationSequence=XYX  RotationSequenceAngles=[0 0 0]  RotationSequenceAnglesUnits=deg  RotationMatrix=[1 0 0; 0 1 0; 0 0 1]
  Transform1 : sm_lib/Frames and Transforms/Rigid Transform  TranslationMethod=Cartesian  TranslationStandardOffset=0  TranslationLengthUnit=mm  TranslationStandardAxis=+Z  TranslationCartesianOffset=smiData.RigidTransform(119).translation  TranslationROffset=0  TranslationROffsetUnits=m  TranslationZOffset=0  TranslationZOffsetUnits=m  TranslationThetaOffset=0  TranslationThetaOffsetUnits=deg  RotationMethod=ArbitraryAxis  RotationAngleUnits=rad  RotationStandardAxis=+Z  RotationAngle=smiData.RigidTransform(119).angle  RotationArbitraryAxis=smiData.RigidTransform(119).axis  FollAlignAxisA=+X  BaseAlignAxisA=+Y  FollAlignAxisB=+Y  BaseAlignAxisB=+Z  RotationSequenceAxes=FollowerAxes  RotationSequence=XYX  RotationSequenceAngles=[0 0 0]  RotationSequenceAnglesUnits=deg  RotationMatrix=[1 0 0; 0 1 0; 0 0 1]
  Transform2 : sm_lib/Frames and Transforms/Rigid Transform  TranslationMethod=Cartesian  TranslationStandardOffset=0  TranslationLengthUnit=mm  TranslationStandardAxis=+Z  TranslationCartesianOffset=smiData.RigidTransform(120).translation  TranslationROffset=0  TranslationROffsetUnits=m  TranslationZOffset=0  TranslationZOffsetUnits=m  TranslationThetaOffset=0  TranslationThetaOffsetUnits=deg  RotationMethod=ArbitraryAxis  RotationAngleUnits=rad  RotationStandardAxis=+Z  RotationAngle=smiData.RigidTransform(120).angle  RotationArbitraryAxis=smiData.RigidTransform(120).axis  FollAlignAxisA=+X  BaseAlignAxisA=+Y  FollAlignAxisB=+Y  BaseAlignAxisB=+Z  RotationSequenceAxes=FollowerAxes  RotationSequence=XYX  RotationSequenceAngles=[0 0 0]  RotationSequenceAnglesUnits=deg  RotationMatrix=[1 0 0; 0 1 0; 0 0 1]
  Transform3 : sm_lib/Frames and Transforms/Rigid Transform  TranslationMethod=Cartesian  TranslationStandardOffset=0  TranslationLengthUnit=mm  TranslationStandardAxis=+Z  TranslationCartesianOffset=smiData.RigidTransform(121).translation  TranslationROffset=0  TranslationROffsetUnits=m  TranslationZOffset=0  TranslationZOffsetUnits=m  TranslationThetaOffset=0  TranslationThetaOffsetUnits=deg  RotationMethod=ArbitraryAxis  RotationAngleUnits=rad  RotationStandardAxis=+Z  RotationAngle=smiData.RigidTransform(121).angle  RotationArbitraryAxis=smiData.RigidTransform(121).axis  FollAlignAxisA=+X  BaseAlignAxisA=+Y  FollAlignAxisB=+Y  BaseAlignAxisB=+Z  RotationSequenceAxes=FollowerAxes  RotationSequence=XYX  RotationSequenceAngles=[0 0 0]  RotationSequenceAnglesUnits=deg  RotationMatrix=[1 0 0; 0 1 0; 0 0 1]
  Transform4 : sm_lib/Frames and Transforms/Rigid Transform  TranslationMethod=Cartesian  TranslationStandardOffset=0  TranslationLengthUnit=mm  TranslationStandardAxis=+Z  TranslationCartesianOffset=smiData.RigidTransform(122).translation  TranslationROffset=0  TranslationROffsetUnits=m  TranslationZOffset=0  TranslationZOffsetUnits=m  TranslationThetaOffset=0  TranslationThetaOffsetUnits=deg  RotationMethod=ArbitraryAxis  RotationAngleUnits=rad  RotationStandardAxis=+Z  RotationAngle=smiData.RigidTransform(122).angle  RotationArbitraryAxis=smiData.RigidTransform(122).axis  FollAlignAxisA=+X  BaseAlignAxisA=+Y  FollAlignAxisB=+Y  BaseAlignAxisB=+Z  RotationSequenceAxes=FollowerAxes  RotationSequence=XYX  RotationSequenceAngles=[0 0 0]  RotationSequenceAnglesUnits=deg  RotationMatrix=[1 0 0; 0 1 0; 0 0 1]
  F : PMIOPort  Side=Right
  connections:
  Resistance_1_RIGID/LConn1 -- Transform/RConn1
  Resistance_3_RIGID/LConn1 -- Transform1/RConn1
  Resistance_2_RIGID/LConn1 -- Transform2/RConn1
  Resistance_4_RIGID/LConn1 -- Transform3/RConn1
  ReferenceFrame/RConn1 -- Transform2/LConn1 -- Transform3/LConn1 -- Transform/LConn1 -- Transform1/LConn1 -- Transform4/RConn1
  Transform4/LConn1 -- F/RConn1

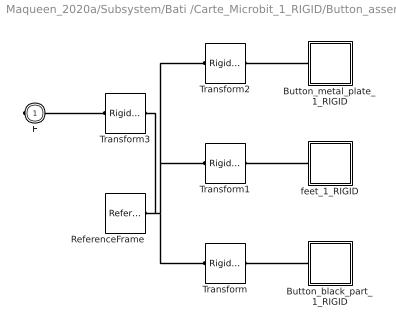
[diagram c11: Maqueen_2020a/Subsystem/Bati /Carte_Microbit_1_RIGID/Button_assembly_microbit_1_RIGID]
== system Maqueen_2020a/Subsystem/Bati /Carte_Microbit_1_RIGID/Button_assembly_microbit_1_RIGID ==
  Button_black_part_1_RIGID : Subsystem
  Button_metal_plate_1_RIGID : Subsystem
  ReferenceFrame : sm_lib/Frames and Transforms/Reference Frame
  Transform : sm_lib/Frames and Transforms/Rigid Transform  TranslationMethod=Cartesian  TranslationStandardOffset=0  TranslationLengthUnit=mm  TranslationStandardAxis=+Z  TranslationCartesianOffset=smiData.RigidTransform(141).translation  TranslationROffset=0  TranslationROffsetUnits=m  TranslationZOffset=0  TranslationZOffsetUnits=m  TranslationThetaOffset=0  TranslationThetaOffsetUnits=deg  RotationMethod=ArbitraryAxis  RotationAngleUnits=rad  RotationStandardAxis=+Z  RotationAngle=smiData.RigidTransform(141).angle  RotationArbitraryAxis=smiData.RigidTransform(141).axis  FollAlignAxisA=+X  BaseAlignAxisA=+Y  FollAlignAxisB=+Y  BaseAlignAxisB=+Z  RotationSequenceAxes=FollowerAxes  RotationSequence=XYX  RotationSequenceAngles=[0 0 0]  RotationSequenceAnglesUnits=deg  RotationMatrix=[1 0 0; 0 1 0; 0 0 1]
  Transform1 : sm_lib/Frames and Transforms/Rigid Transform  TranslationMethod=Cartesian  TranslationStandardOffset=0  TranslationLengthUnit=mm  TranslationStandardAxis=+Z  TranslationCartesianOffset=smiData.RigidTransform(142).translation  TranslationROffset=0  TranslationROffsetUnits=m  TranslationZOffset=0  TranslationZOffsetUnits=m  TranslationThetaOffset=0  TranslationThetaOffsetUnits=deg  RotationMethod=ArbitraryAxis  RotationAngleUnits=rad  RotationStandardAxis=+Z  RotationAngle=smiData.RigidTransform(142).angle  RotationArbitraryAxis=smiData.RigidTransform(142).axis  FollAlignAxisA=+X  BaseAlignAxisA=+Y  FollAlignAxisB=+Y  BaseAlignAxisB=+Z  RotationSequenceAxes=FollowerAxes  RotationSequence=XYX  RotationSequenceAngles=[0 0 0]  RotationSequenceAnglesUnits=deg  RotationMatrix=[1 0 0; 0 1 0; 0 0 1]
  Transform2 : sm_lib/Frames and Transforms/Rigid Transform  TranslationMethod=Cartesian  TranslationStandardOffset=0  TranslationLengthUnit=mm  TranslationStandardAxis=+Z  TranslationCartesianOffset=smiData.RigidTransform(143).translation  TranslationROffset=0  TranslationROffsetUnits=m  TranslationZOffset=0  TranslationZOffsetUnits=m  TranslationThetaOffset=0  TranslationThetaOffsetUnits=deg  RotationMethod=ArbitraryAxis  RotationAngleUnits=rad  RotationStandardAxis=+Z  RotationAngle=smiData.RigidTransform(143).angle  RotationArbitraryAxis=smiData.RigidTransform(143).axis  FollAlignAxisA=+X  BaseAlignAxisA=+Y  FollAlignAxisB=+Y  BaseAlignAxisB=+Z  RotationSequenceAxes=FollowerAxes  RotationSequence=XYX  RotationSequenceAngles=[0 0 0]  RotationSequenceAnglesUnits=deg  RotationMatrix=[1 0 0; 0 1 0; 0 0 1]
  Transform3 : sm_lib/Frames and Transforms/Rigid Transform  TranslationMethod=Cartesian  TranslationStandardOffset=0  TranslationLengthUnit=mm  TranslationStandardAxis=+Z  TranslationCartesianOffset=smiData.RigidTransform(144).translation  TranslationROffset=0  TranslationROffsetUnits=m  TranslationZOffset=0  TranslationZOffsetUnits=m  TranslationThetaOffset=0  TranslationThetaOffsetUnits=deg  RotationMethod=ArbitraryAxis  RotationAngleUnits=rad  RotationStandardAxis=+Z  RotationAngle=smiData.RigidTransform(144).angle  RotationArbitraryAxis=smiData.RigidTransform(144).axis  FollAlignAxisA=+X  BaseAlignAxisA=+Y  FollAlignAxisB=+Y  BaseAlignAxisB=+Z  RotationSequenceAxes=FollowerAxes  RotationSequence=XYX  RotationSequenceAngles=[0 0 0]  RotationSequenceAnglesUnits=deg  RotationMatrix=[1 0 0; 0 1 0; 0 0 1]
  feet_1_RIGID : Subsystem
  F : PMIOPort  Side=Right
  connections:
  Button_black_part_1_RIGID/LConn1 -- Transform/RConn1
  Transform1/RConn1 -- feet_1_RIGID/LConn1
  Button_metal_plate_1_RIGID/LConn1 -- Transform2/RConn1
  ReferenceFrame/RConn1 -- Transform1/LConn1 -- Transform2/LConn1 -- Transform/LConn1 -- Transform3/RConn1
  Transform3/LConn1 -- F/RConn1

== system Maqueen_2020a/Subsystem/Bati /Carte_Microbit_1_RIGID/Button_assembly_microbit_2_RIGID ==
  Button_black_part_1_RIGID : Subsystem
  Button_metal_plate_1_RIGID : Subsystem
  ReferenceFrame : sm_lib/Frames and Transforms/Reference Frame
  Transform : sm_lib/Frames and Transforms/Rigid Transform  TranslationMethod=Cartesian  TranslationStandardOffset=0  TranslationLengthUnit=mm  TranslationStandardAxis=+Z  TranslationCartesianOffset=smiData.RigidTransform(130).translation  TranslationROffset=0  TranslationROffsetUnits=m  TranslationZOffset=0  TranslationZOffsetUnits=m  TranslationThetaOffset=0  TranslationThetaOffsetUnits=deg  RotationMethod=ArbitraryAxis  RotationAngleUnits=rad  RotationStandardAxis=+Z  RotationAngle=smiData.RigidTransform(130).angle  RotationArbitraryAxis=smiData.RigidTransform(130).axis  FollAlignAxisA=+X  BaseAlignAxisA=+Y  FollAlignAxisB=+Y  BaseAlignAxisB=+Z  RotationSequenceAxes=FollowerAxes  RotationSequence=XYX  RotationSequenceAngles=[0 0 0]  RotationSequenceAnglesUnits=deg  RotationMatrix=[1 0 0; 0 1 0; 0 0 1]
  Transform1 : sm_lib/Frames and Transforms/Rigid Transform  TranslationMethod=Cartesian  TranslationStandardOffset=0  TranslationLengthUnit=mm  TranslationStandardAxis=+Z  TranslationCartesianOffset=smiData.RigidTransform(131).translation  TranslationROffset=0  TranslationROffsetUnits=m  TranslationZOffset=0  TranslationZOffsetUnits=m  TranslationThetaOffset=0  TranslationThetaOffsetUnits=deg  RotationMethod=ArbitraryAxis  RotationAngleUnits=rad  RotationStandardAxis=+Z  RotationAngle=smiData.RigidTransform(131).angle  RotationArbitraryAxis=smiData.RigidTransform(131).axis  FollAlignAxisA=+X  BaseAlignAxisA=+Y  FollAlignAxisB=+Y  BaseAlignAxisB=+Z  RotationSequenceAxes=FollowerAxes  RotationSequence=XYX  RotationSequenceAngles=[0 0 0]  RotationSequenceAnglesUnits=deg  RotationMatrix=[1 0 0; 0 1 0; 0 0 1]
  Transform2 : sm_lib/Frames and Transforms/Rigid Transform  TranslationMethod=Cartesian  TranslationStandardOffset=0  TranslationLengthUnit=mm  TranslationStandardAxis=+Z  TranslationCartesianOffset=smiData.RigidTransform(132).translation  TranslationROffset=0  TranslationROffsetUnits=m  TranslationZOffset=0  TranslationZOffsetUnits=m  TranslationThetaOffset=0  TranslationThetaOffsetUnits=deg  RotationMethod=ArbitraryAxis  RotationAngleUnits=rad  RotationStandardAxis=+Z  RotationAngle=smiData.RigidTransform(132).angle  RotationArbitraryAxis=smiData.RigidTransform(132).axis  FollAlignAxisA=+X  BaseAlignAxisA=+Y  FollAlignAxisB=+Y  BaseAlignAxisB=+Z  RotationSequenceAxes=FollowerAxes  RotationSequence=XYX  RotationSequenceAngles=[0 0 0]  RotationSequenceAnglesUnits=deg  RotationMatrix=[1 0 0; 0 1 0; 0 0 1]
  Transform3 : sm_lib/Frames and Transforms/Rigid Transform  TranslationMethod=Cartesian  TranslationStandardOffset=0  TranslationLengthUnit=mm  TranslationStandardAxis=+Z  TranslationCartesianOffset=smiData.RigidTransform(133).translation  TranslationROffset=0  TranslationROffsetUnits=m  TranslationZOffset=0  TranslationZOffsetUnits=m  TranslationThetaOffset=0  TranslationThetaOffsetUnits=deg  RotationMethod=ArbitraryAxis  RotationAngleUnits=rad  RotationStandardAxis=+Z  RotationAngle=smiData.RigidTransform(133).angle  RotationArbitraryAxis=smiData.RigidTransform(133).axis  FollAlignAxisA=+X  BaseAlignAxisA=+Y  FollAlignAxisB=+Y  BaseAlignAxisB=+Z  RotationSequenceAxes=FollowerAxes  RotationSequence=XYX  RotationSequenceAngles=[0 0 0]  RotationSequenceAnglesUnits=deg  RotationMatrix=[1 0 0; 0 1 0; 0 0 1]
  feet_1_RIGID : Subsystem
  F : PMIOPort  Side=Right
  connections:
  Button_black_part_1_RIGID/LConn1 -- Transform/RConn1
  Transform1/RConn1 -- feet_1_RIGID/LConn1
  Button_metal_plate_1_RIGID/LConn1 -- Transform2/RConn1
  ReferenceFrame/RConn1 -- Transform1/LConn1 -- Transform2/LConn1 -- Transform/LConn1 -- Transform3/RConn1
  Transform3/LConn1 -- F/RConn1

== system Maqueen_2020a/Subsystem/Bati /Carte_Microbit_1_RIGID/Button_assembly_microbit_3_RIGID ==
  Button_black_part_1_RIGID : Subsystem
  Button_metal_plate_1_RIGID : Subsystem
  ReferenceFrame : sm_lib/Frames and Transforms/Reference Frame
  Transform : sm_lib/Frames and Transforms/Rigid Transform  TranslationMethod=Cartesian  TranslationStandardOffset=0  TranslationLengthUnit=mm  TranslationStandardAxis=+Z  TranslationCartesianOffset=smiData.RigidTransform(146).translation  TranslationROffset=0  TranslationROffsetUnits=m  TranslationZOffset=0  TranslationZOffsetUnits=m  TranslationThetaOffset=0  TranslationThetaOffsetUnits=deg  RotationMethod=ArbitraryAxis  RotationAngleUnits=rad  RotationStandardAxis=+Z  RotationAngle=smiData.RigidTransform(146).angle  RotationArbitraryAxis=smiData.RigidTransform(146).axis  FollAlignAxisA=+X  BaseAlignAxisA=+Y  FollAlignAxisB=+Y  BaseAlignAxisB=+Z  RotationSequenceAxes=FollowerAxes  RotationSequence=XYX  RotationSequenceAngles=[0 0 0]  RotationSequenceAnglesUnits=deg  RotationMatrix=[1 0 0; 0 1 0; 0 0 1]
  Transform1 : sm_lib/Frames and Transforms/Rigid Transform  TranslationMethod=Cartesian  TranslationStandardOffset=0  TranslationLengthUnit=mm  TranslationStandardAxis=+Z  TranslationCartesianOffset=smiData.RigidTransform(147).translation  TranslationROffset=0  TranslationROffsetUnits=m  TranslationZOffset=0  TranslationZOffsetUnits=m  TranslationThetaOffset=0  TranslationThetaOffsetUnits=deg  RotationMethod=ArbitraryAxis  RotationAngleUnits=rad  RotationStandardAxis=+Z  RotationAngle=smiData.RigidTransform(147).angle  RotationArbitraryAxis=smiData.RigidTransform(147).axis  FollAlignAxisA=+X  BaseAlignAxisA=+Y  FollAlignAxisB=+Y  BaseAlignAxisB=+Z  RotationSequenceAxes=FollowerAxes  RotationSequence=XYX  RotationSequenceAngles=[0 0 0]  RotationSequenceAnglesUnits=deg  RotationMatrix=[1 0 0; 0 1 0; 0 0 1]
  Transform2 : sm_lib/Frames and Transforms/Rigid Transform  TranslationMethod=Cartesian  TranslationStandardOffset=0  TranslationLengthUnit=mm  TranslationStandardAxis=+Z  TranslationCartesianOffset=smiData.RigidTransform(148).translation  TranslationROffset=0  TranslationROffsetUnits=m  TranslationZOffset=0  TranslationZOffsetUnits=m  TranslationThetaOffset=0  TranslationThetaOffsetUnits=deg  RotationMethod=ArbitraryAxis  RotationAngleUnits=rad  RotationStandardAxis=+Z  RotationAngle=smiData.RigidTransform(148).angle  RotationArbitraryAxis=smiData.RigidTransform(148).axis  FollAlignAxisA=+X  BaseAlignAxisA=+Y  FollAlignAxisB=+Y  BaseAlignAxisB=+Z  RotationSequenceAxes=FollowerAxes  RotationSequence=XYX  RotationSequenceAngles=[0 0 0]  RotationSequenceAnglesUnits=deg  RotationMatrix=[1 0 0; 0 1 0; 0 0 1]
  Transform3 : sm_lib/Frames and Transforms/Rigid Transform  TranslationMethod=Cartesian  TranslationStandardOffset=0  TranslationLengthUnit=mm  TranslationStandardAxis=+Z  TranslationCartesianOffset=smiData.RigidTransform(149).translation  TranslationROffset=0  TranslationROffsetUnits=m  TranslationZOffset=0  TranslationZOffsetUnits=m  TranslationThetaOffset=0  TranslationThetaOffsetUnits=deg  RotationMethod=ArbitraryAxis  RotationAngleUnits=rad  RotationStandardAxis=+Z  RotationAngle=smiData.RigidTransform(149).angle  RotationArbitraryAxis=smiData.RigidTransform(149).axis  FollAlignAxisA=+X  BaseAlignAxisA=+Y  FollAlignAxisB=+Y  BaseAlignAxisB=+Z  RotationSequenceAxes=FollowerAxes  RotationSequence=XYX  RotationSequenceAngles=[0 0 0]  RotationSequenceAnglesUnits=deg  RotationMatrix=[1 0 0; 0 1 0; 0 0 1]
  feet_1_RIGID : Subsystem
  F : PMIOPort  Side=Right
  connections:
  Button_black_part_1_RIGID/LConn1 -- Transform/RConn1
  Transform1/RConn1 -- feet_1_RIGID/LConn1
  Button_metal_plate_1_RIGID/LConn1 -- Transform2/RConn1
  ReferenceFrame/RConn1 -- Transform1/LConn1 -- Transform2/LConn1 -- Transform/LConn1 -- Transform3/RConn1
  Transform3/LConn1 -- F/RConn1

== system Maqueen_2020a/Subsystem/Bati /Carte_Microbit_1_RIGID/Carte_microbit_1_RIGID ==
  ReferenceFrame : sm_lib/Frames and Transforms/Reference Frame
  Solid : sm_lib/Body Elements/File Solid  ExtGeomFileName=Carte microbit_Defaut_sldprt.STL  UnitType=Custom  ExtGeomFileUnits=mm  StepReaderType=HEX  ExportConvexHullGeometry=off  InertiaType=Custom  Mass=smiData.Solid(26).mass  MassUnits=kg  CenterOfMass=smiData.Solid(26).CoM  CenterOfMassUnits=mm  MomentsOfInertia=smiData.Solid(26).MoI  MomentsOfInertiaUnits=kg*mm^2  ProductsOfInertia=smiData.Solid(26).PoI  ProductsOfInertiaUnits=kg*mm^2  BasedOnType=Density  Density=1000  DensityUnits=kg/m^3  DoExposeReferenceFrame=on  SerializedFrames=<Frames/>  GraphicType=FromGeometry  MarkerShape=Sphere  MarkerSize=10  GraphicVisPropType=SimpleVisualProperties  GraphicDiffuseColor=smiData.Solid(26).color  GraphicSpecularColor=[0.5 0.5 0.5 1.0]  GraphicAmbientColor=[0.15 0.15 0.15 1.0]  GraphicEmissiveColor=[0.0 0.0 0.0 1.0]  GraphicShininess=75  GraphicOpacity=smiData.Solid(26).opacity
  F : PMIOPort  Side=Left
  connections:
  ReferenceFrame/RConn1 -- Solid/RConn1 -- F/RConn1

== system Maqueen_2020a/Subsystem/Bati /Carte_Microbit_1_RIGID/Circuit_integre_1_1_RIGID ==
  ReferenceFrame : sm_lib/Frames and Transforms/Reference Frame
  Solid : sm_lib/Body Elements/File Solid  ExtGeomFileName=Circuit integre 1_Defaut_sldprt.STL  UnitType=Custom  ExtGeomFileUnits=mm  StepReaderType=HEX  ExportConvexHullGeometry=off  InertiaType=Custom  Mass=smiData.Solid(11).mass  MassUnits=kg  CenterOfMass=smiData.Solid(11).CoM  CenterOfMassUnits=mm  MomentsOfInertia=smiData.Solid(11).MoI  MomentsOfInertiaUnits=kg*mm^2  ProductsOfInertia=smiData.Solid(11).PoI  ProductsOfInertiaUnits=kg*mm^2  BasedOnType=Density  Density=1000  DensityUnits=kg/m^3  DoExposeReferenceFrame=on  SerializedFrames=<Frames/>  GraphicType=FromGeometry  MarkerShape=Sphere  MarkerSize=10  GraphicVisPropType=SimpleVisualProperties  GraphicDiffuseColor=smiData.Solid(11).color  GraphicSpecularColor=[0.5 0.5 0.5 1.0]  GraphicAmbientColor=[0.15 0.15 0.15 1.0]  GraphicEmissiveColor=[0.0 0.0 0.0 1.0]  GraphicShininess=75  GraphicOpacity=smiData.Solid(11).opacity
  F : PMIOPort  Side=Left
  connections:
  ReferenceFrame/RConn1 -- Solid/RConn1 -- F/RConn1
